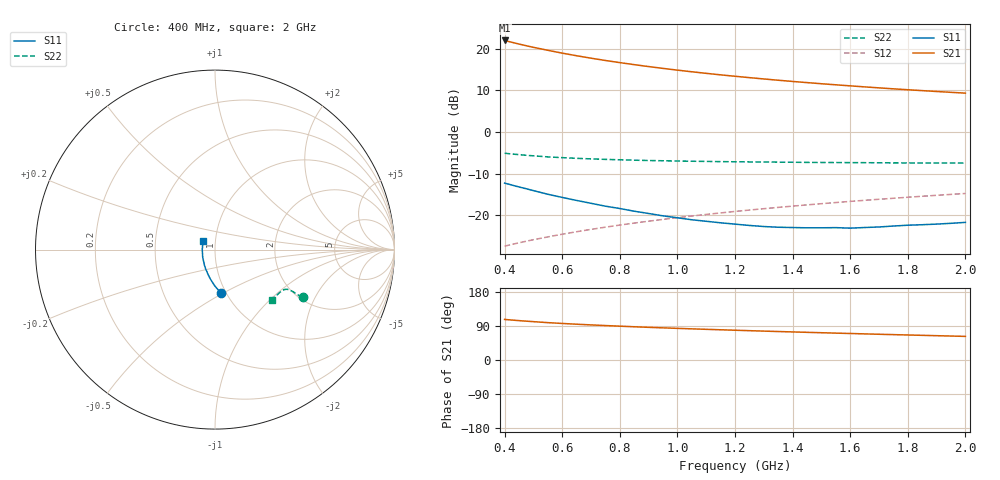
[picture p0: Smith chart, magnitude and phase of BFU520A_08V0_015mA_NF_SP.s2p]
! Filename:  P:\Prog\Test\Noise\ATS_data\Testdata_Net\06 Compressed Noise after Statistics\BFU520A_APG2013_30_A05_08p0V_015mA_NF_CM01_D.sf
! Date/Time: Wed 24/Apr/2013 20:06:20
! BFU520A_APG2013_30_A05_08p0V_1to20mA_NF_CM01_Bias7_R.sf
! Noise Parameter Data File
! BFU520A_APG2013_30_A05_08p0V_1to20mA_NF_CM01
! Date/time: Thu Apr 11 09:33:54 2013
! VAR V_out= 8.000000
! VAR I_out= 14.990000
! VAR V_in= 0.829600
! VAR I_in= 0.161450
! Device data file deembeded for feedlines and parallel
! Original file: \06 Compressed Noise after Statistics\BFU520A_APG2013_30_A05_08p0V_015mA_NF_CM01_R.sf
! Feed-files: PR017V01_150413_Feed1.s2p, PR017V01_150413_Feed2.s2p
! Parallel-file: PR017V01_150413_Par.s2p
# MHz S MA R 50
!  Freq-MHz  S11-mag  S11-arg  S21-mag  S21-arg  S12-mag  S12-arg  S22-mag  S22-arg
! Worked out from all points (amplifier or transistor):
!   37 points, 400 MHz to 2 GHz, reference 50 ohm
!   highest |S21| = 21.9 dB at 400 MHz (marker M1)
!   |S21| within 3 dB of that: start of sweep to 597 MHz
!   unconditionally stable (mu >= 1): 1.141 GHz to end of sweep
!   at 500 MHz: K = 0.89, MSG = 23.1 dB, |S12| = -25.8 dB
!   at 1.1 GHz: K = 1.00, MSG = 16.9 dB, |S12| = -19.8 dB
!   at 2 GHz: K = 1.00, MAG = 12.0 dB, |S12| = -14.8 dB
!   lowest NFmin = 1.01 dB at 420 MHz
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400  0.2435 -81.8  12.51 107.1  0.0427 72.0  0.5557 -28.7
420  0.2335 -83.8  12.01 105.7  0.04436 72.1  0.5463 -28.7
440  0.2236 -85.8  11.55 104.5  0.04603 72.2  0.5382 -28.6
460  0.2148 -87.5  11.12 103.3  0.04769 72.4  0.5309 -28.6
480  0.2066 -89.3  10.72 102.2  0.04934 72.5  0.5233 -28.6
500  0.198 -91.2  10.35 101.2  0.05103 72.6  0.5173 -28.6
550  0.179 -95.4  9.539 98.6  0.05514 73.0  0.5024 -28.4
600  0.1641 -99.5  8.815 96.4  0.05939 73.2  0.4921 -28.3
650  0.1509 -103.2  8.205 94.5  0.06361 73.4  0.4829 -28.4
700  0.1395 -107.2  7.67 92.6  0.06786 73.6  0.4755 -28.4
750  0.1288 -111.0  7.197 90.9  0.07216 73.8  0.469 -28.5
800  0.1208 -115.3  6.785 89.3  0.07645 73.8  0.4636 -28.6
850  0.1121 -119.5  6.416 87.7  0.08077 73.8  0.4588 -28.9
950  0.0986 -128.0  5.784 84.8  0.08941 73.9  0.4513 -29.4
1050  0.08851 -136.8  5.269 82.2  0.09812 73.8  0.4455 -30.0
1150  0.08139 -146.8  4.841 79.8  0.1069 73.5  0.4408 -30.8
1200  0.07847 -151.1  4.654 78.6  0.1114 73.4  0.439 -31.3
1350  0.07202 -165.9  4.171 75.1  0.1246 72.9  0.4346 -32.8
1500  0.07091 179.2  3.787 72.0  0.1379 72.3  0.4304 -34.5
1650  0.07146 166.6  3.472 68.9  0.1515 71.5  0.4282 -36.4
1750  0.07447 158.8  3.289 67.0  0.1603 71.0  0.4258 -37.7
2000  0.08237 143.3  2.921 62.3  0.1829 69.5  0.4231 -41.3
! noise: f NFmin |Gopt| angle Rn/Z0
400  1.042  0.112  -166.2  0.1064
460  1.024  0.1225  -165.4  0.0979
600  1.129  0.1207  -158.4  0.1134
800  1.079  0.1536  -158  0.0942
1000  1.102  0.1623  -150  0.0977
1200  1.144  0.1761  -143.1  0.1022
1400  1.16  0.1969  -136.7  0.1066
1600  1.166  0.2049  -129.9  0.1097
1800  1.126  0.2264  -126.3  0.1159
2000  1.215  0.2392  -120.7  0.1147
